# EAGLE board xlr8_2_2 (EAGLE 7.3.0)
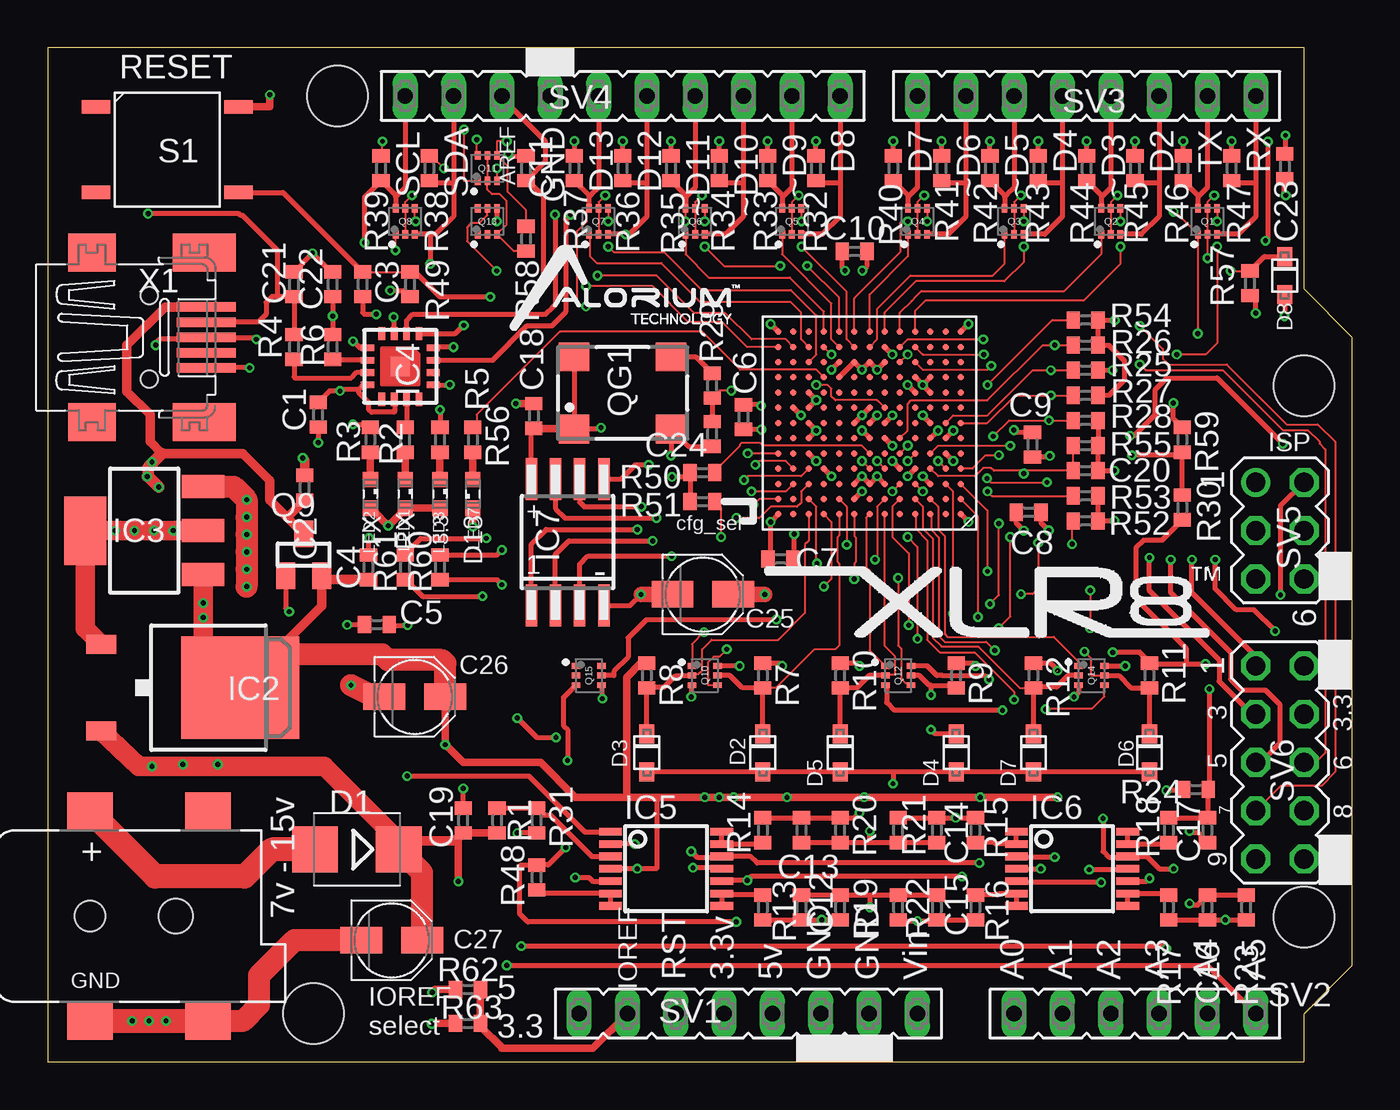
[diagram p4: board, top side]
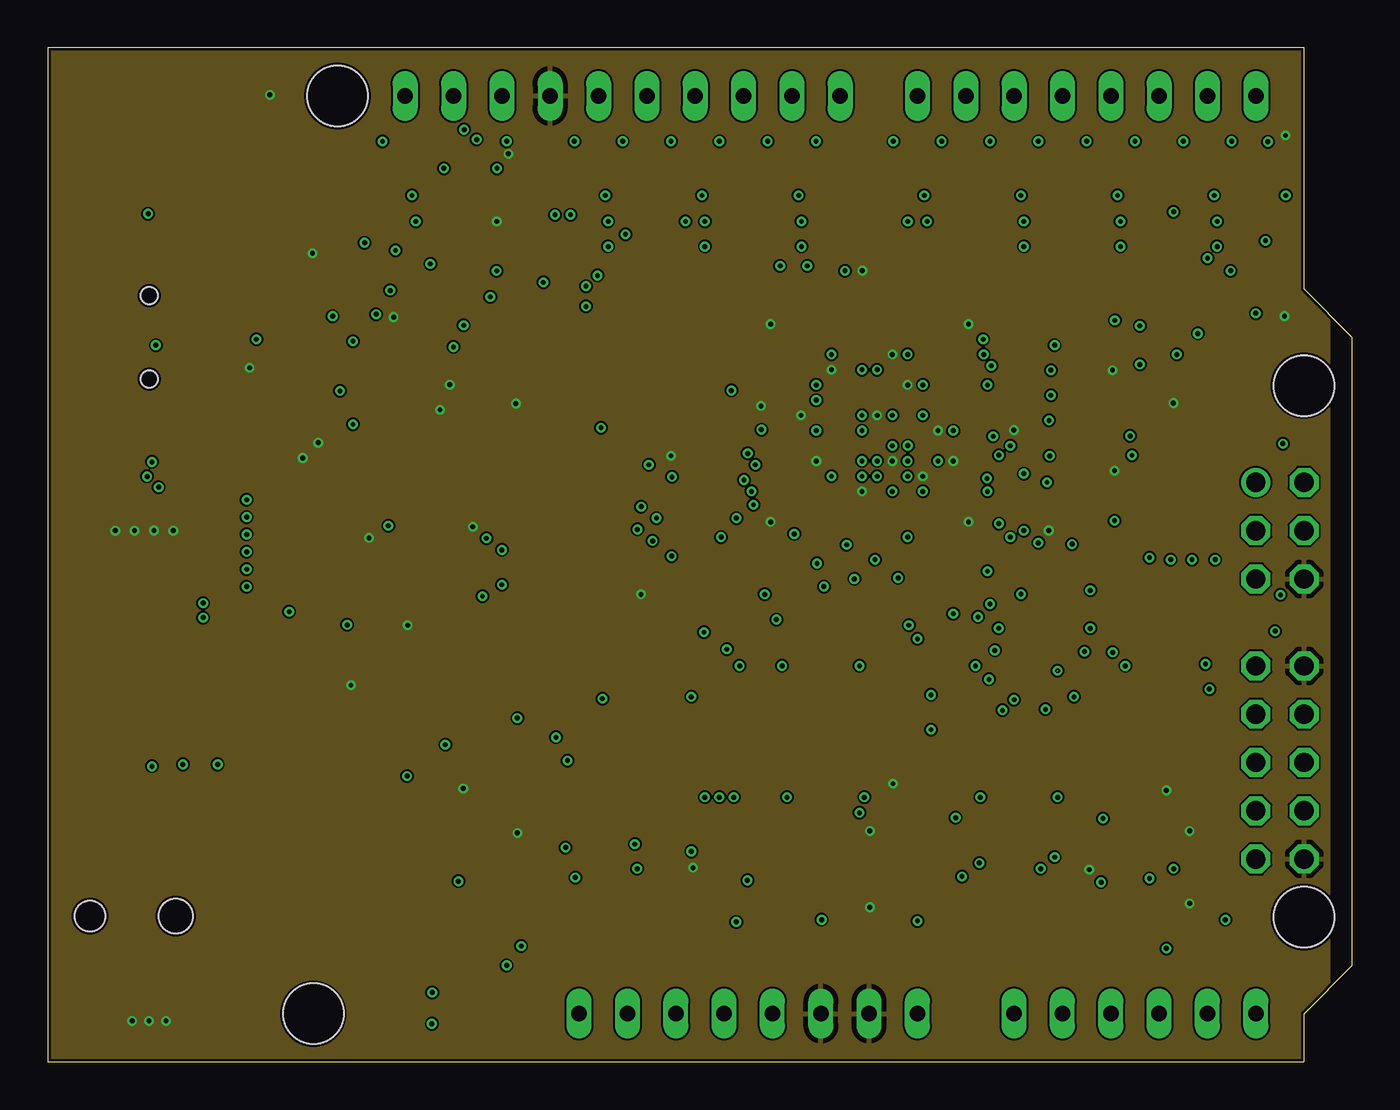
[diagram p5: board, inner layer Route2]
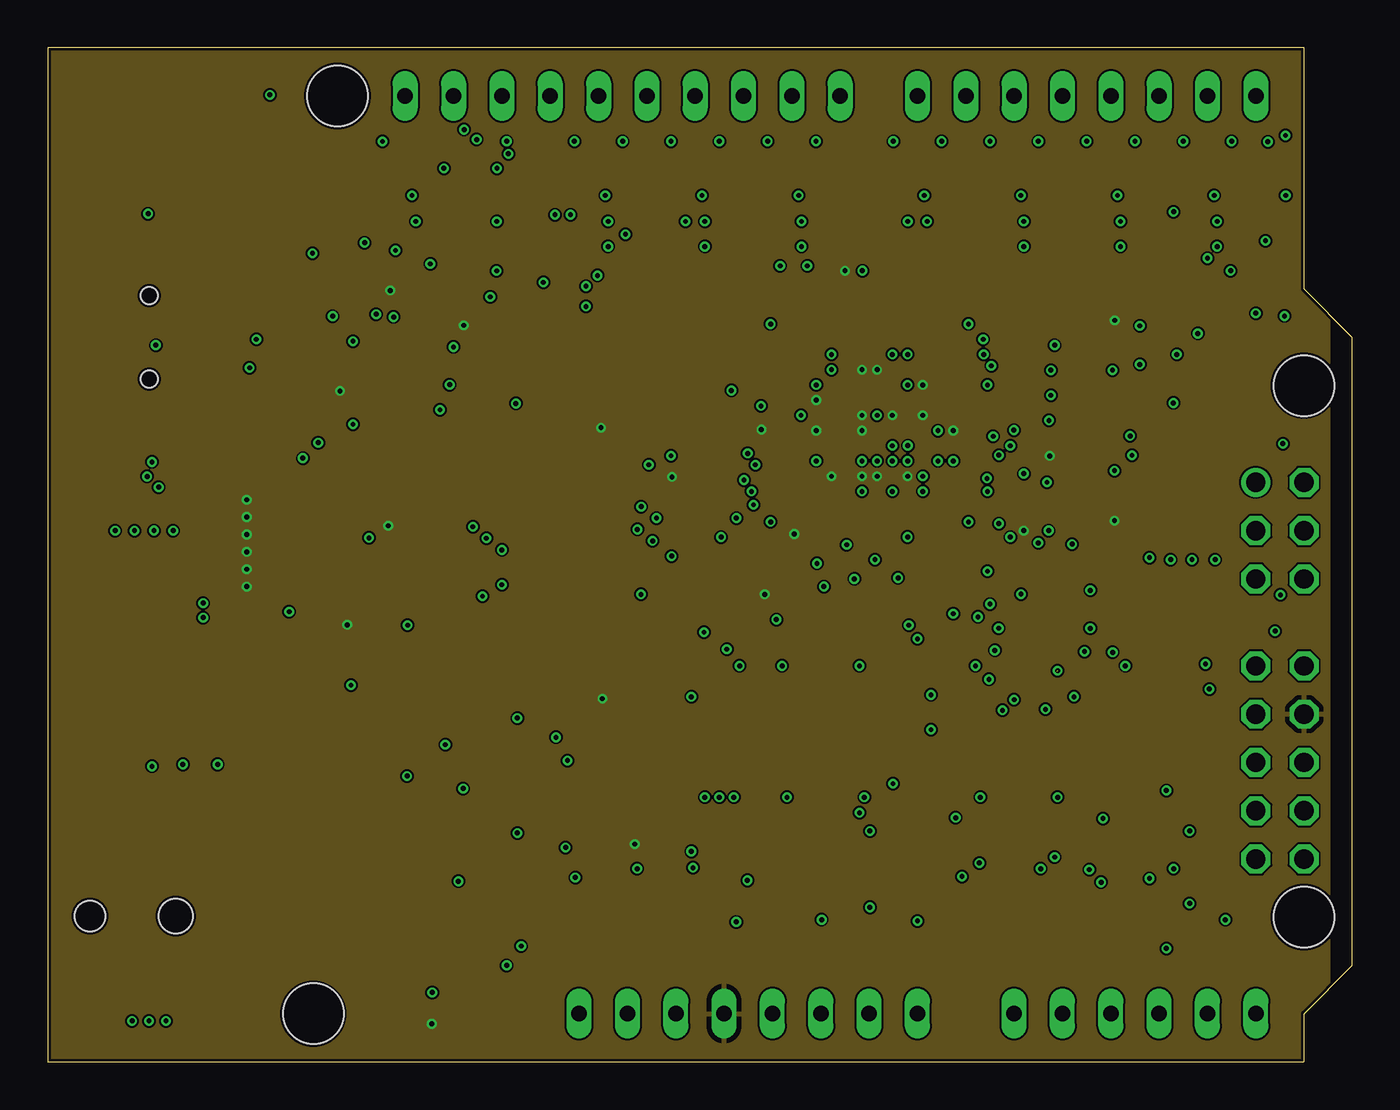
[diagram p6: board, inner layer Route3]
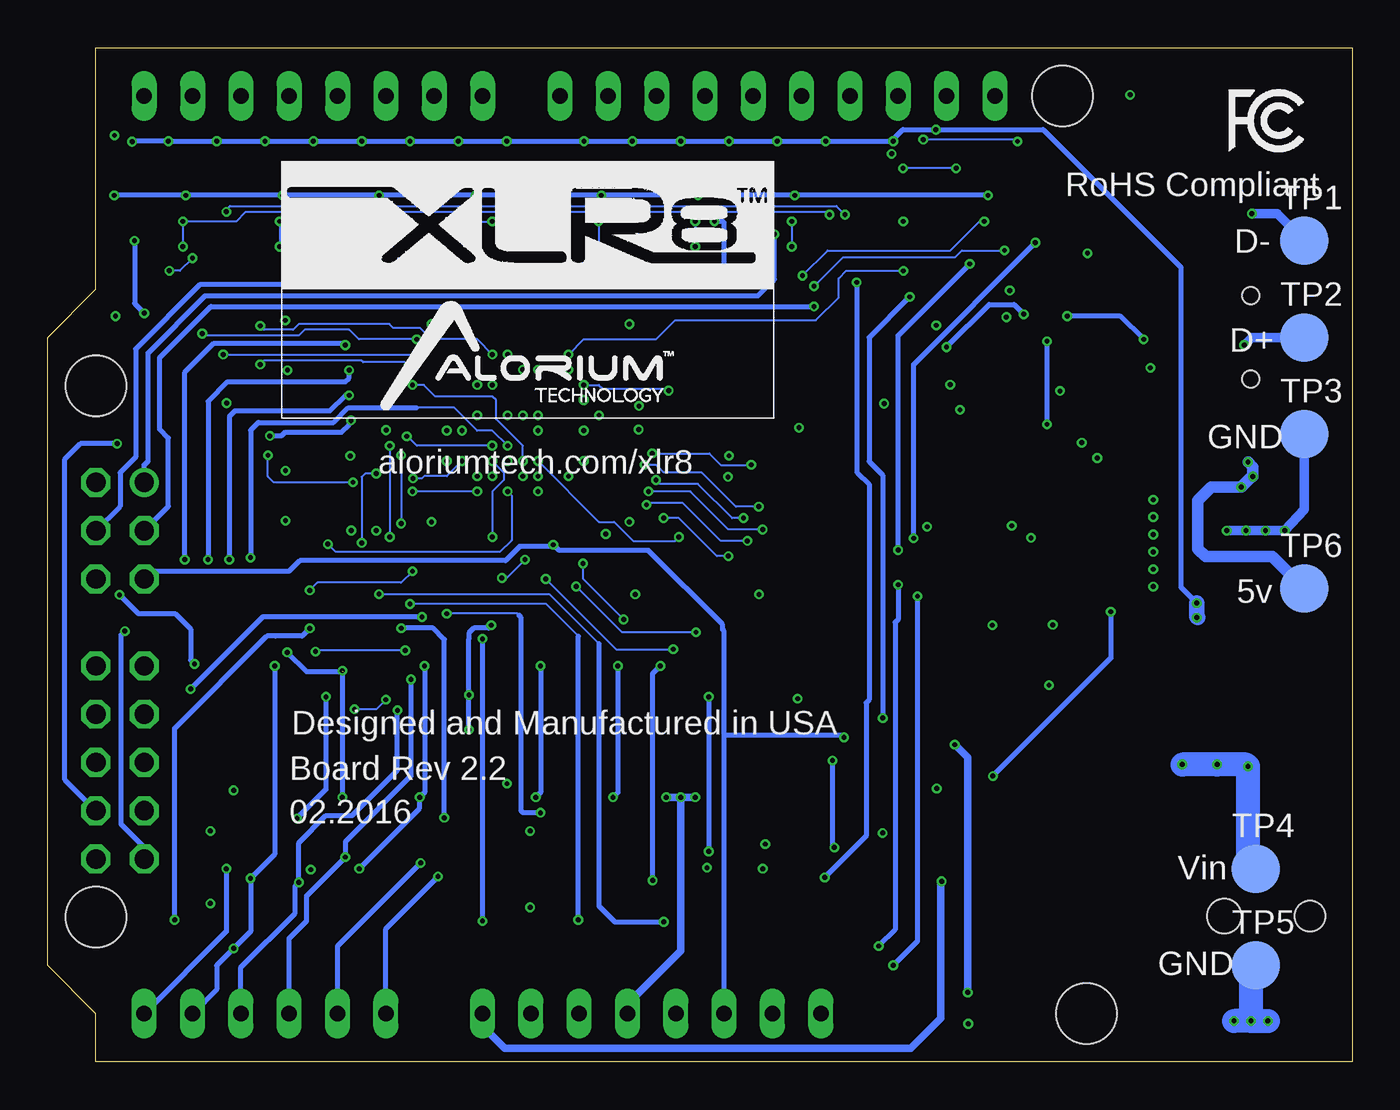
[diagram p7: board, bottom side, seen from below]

Size 68.58 x 53.34 mm. Coordinates in mm from the lower left corner, seen from the top.
Outline: 66.02,0 0,0 0,53.34 66.04,53.34 66.04,40.64 68.58,38.1 68.58,5.08 66.04,2.54 66.04,0
Copper layers (1*2*3*16): Top 0.035mm / dielectric 0.204mm / Route2 0.035mm / dielectric 0.252mm / Route3 0.035mm / dielectric 0.204mm / Bottom 0.035mm
Design rules "default *": minimum track width 4mil, minimum drill 10mil, track to track 4mil, track to pad 5mil, pad to pad 6mil, via to via 6mil, smd to smd 6mil, copper to edge 6mil, drill to drill 6mil, minimum pad ring 10mil, minimum via ring 5mil, stop-mask expansion 0mil, vias tented up to drill 25mil, thermal gap 10mil
Holes 3.17 mm at 15.24,50.8 66.04,7.62 66.04,35.56 13.97,2.54

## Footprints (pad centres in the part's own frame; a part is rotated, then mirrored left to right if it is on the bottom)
C0402 = smd 0.7 x 0.9: 1 -0.65,0; 2 0.65,0
PANASONIC_B = smd 2.2 x 1.4: + 1.6,0; - -1.6,0
DCJACK_2MM_SMT = smd 2.4 x 2: GND 0,-5.5; GNDBREAK 6.2,-5.5; PWR1 0,5.5; PWR2 6.2,5.5 | hole 1.6: 0,0 | hole 1.8: 4.5,0
SMB = smd 2.4 x 2.4: A 2.2,0; C -2.2,0
SOD-323F = smd 1 x 0.8: A -1,0; C 1,0
DPACK = smd 1 x 1.6: 1 -2.28,-4.8; 3 2.28,-4.8 | smd 5.4 x 6.2: 2 0,2.5
SOT223 = smd 1.219 x 2.235: 1 -2.311,-3.099; 2 0,-3.099; 3 2.311,-3.099 | smd 3.6 x 2.2: 4 0,3.099
QFN16 = smd 0.7 x 0.35: 1 -1.725,0.975; 2 -1.725,0.325; 3 -1.725,-0.325; 4 -1.725,-0.975; 9 1.725,-0.975; 10 1.725,-0.325; 11 1.725,0.325; 12 1.725,0.975 | smd 0.35 x 0.7: 5 -0.975,-1.725; 6 -0.325,-1.725; 7 0.325,-1.725; 8 0.975,-1.725; 13 0.975,1.725; 14 0.325,1.725; 15 -0.325,1.725; 16 -0.975,1.725 | smd 1 x 1: TAB 0,0
SSOP14 = smd 0.4 x 1.2: 1 -1.95,-2.925; 2 -1.3,-2.925; 3 -0.65,-2.925; 4 0,-2.925; 5 0.65,-2.925; 6 1.3,-2.925; 7 1.95,-2.925; 8 1.95,2.925; 9 1.3,2.925; 10 0.65,2.925; 11 0,2.925; 12 -0.65,2.925; 13 -1.3,2.925; 14 -1.95,2.925
SO-08M = smd 0.6 x 2.2: 1 -1.905,-3.33; 2 -0.635,-3.33; 3 0.635,-3.33; 4 1.905,-3.33; 5 1.905,3.33; 6 0.635,3.33; 7 -0.635,3.33; 8 -1.905,3.33
LED_SML0603 = smd 0.8 x 0.8: A 0.75,0; C -0.75,0
SOT-563 = smd 0.3 x 0.45: 1 -0.5,-0.674; 2 0,-0.674; 3 0.5,-0.674; 4 0.5,0.674; 5 0,0.674; 6 -0.5,0.674
SUPER-SOT3 = smd 1 x 1.4: 1 -0.95,-1.1; 2 0.95,-1.1; 3 0,1.1
SM77H = smd 1.6 x 1.5: 1 -2.55,-1.9; 2 2.55,-1.9; 3 2.55,1.9; 4 -2.55,1.9
R0402 = smd 0.7 x 0.9: 1 -0.65,0; 2 0.65,0
6MM_SMT = smd 1.5 x 0.7: 1 0,4.5; 2 7.5,4.5; 3 0,0; 4 7.5,0
FE08 = drill 0.813 long: 1 -8.89,0; 2 -6.35,0; 3 -3.81,0; 4 -1.27,0; 5 1.27,0; 6 3.81,0; 7 6.35,0; 8 8.89,0
FE06 = drill 0.813 long: 1 -6.35,0; 2 -3.81,0; 3 -1.27,0; 4 1.27,0; 5 3.81,0; 6 6.35,0
FE10 = drill 0.813 long: 1 -11.43,0; 2 -8.89,0; 3 -6.35,0; 4 -3.81,0; 5 -1.27,0; 6 1.27,0; 7 3.81,0; 8 6.35,0; 9 8.89,0; 10 11.43,0
MA03-2 = drill 1.016: 1 -2.54,-1.27 | drill 1.016 octagon: 2 -2.54,1.27; 3 0,-1.27; 4 0,1.27; 5 2.54,-1.27; 6 2.54,1.27
MA05-2 = drill 1.016 octagon: 1 -5.08,-1.27; 2 -5.08,1.27; 3 -2.54,-1.27; 4 -2.54,1.27; 5 0,-1.27; 6 0,1.27; 7 2.54,-1.27; 8 2.54,1.27; 9 5.08,-1.27; 10 5.08,1.27
B2,54 = smd 2.54 x 2.54: TP 0,0
UBGA_169 = smd 0.34 x 0.34: A1 -9.6,0; A2 -8.8,0; A3 -8,0; A4 -7.2,0; A5 -6.4,0; A6 -5.6,0; A7 -4.8,0; A8 -4,0; A9 -3.2,0; A10 -2.4,0; A11 -1.6,0; A12 -0.8,0; A13 0,0; B1 -9.6,-0.8; B2 -8.8,-0.8; B3 -8,-0.8; B4 -7.2,-0.8; B5 -6.4,-0.8; B6 -5.6,-0.8; B7 -4.8,-0.8; B8 -4,-0.8; B9 -3.2,-0.8; B10 -2.4,-0.8; B11 -1.6,-0.8; B12 -0.8,-0.8; B13 0,-0.8; C1 -9.6,-1.6; C2 -8.8,-1.6; C3 -8,-1.6; C4 -7.2,-1.6; C5 -6.4,-1.6; C6 -5.6,-1.6; C7 -4.8,-1.6; C8 -4,-1.6; C9 -3.2,-1.6; C10 -2.4,-1.6; C11 -1.6,-1.6; C12 -0.8,-1.6; C13 0,-1.6; D1 -9.6,-2.4; D2 -8.8,-2.4; D3 -8,-2.4; D4 -7.2,-2.4; D5 -6.4,-2.4; D6 -5.6,-2.4; D7 -4.8,-2.4; D8 -4,-2.4; D9 -3.2,-2.4; D10 -2.4,-2.4; D11 -1.6,-2.4; D12 -0.8,-2.4; D13 0,-2.4; E1 -9.6,-3.2; E2 -8.8,-3.2; E3 -8,-3.2; E4 -7.2,-3.2; E5 -6.4,-3.2; E6 -5.6,-3.2; E7 -4.8,-3.2; E8 -4,-3.2; E9 -3.2,-3.2; E10 -2.4,-3.2; E11 -1.6,-3.2; E12 -0.8,-3.2; E13 0,-3.2; F1 -9.6,-4; F2 -8.8,-4; F3 -8,-4; F4 -7.2,-4; F5 -6.4,-4; F6 -5.6,-4; F7 -4.8,-4; F8 -4,-4; F9 -3.2,-4; F10 -2.4,-4; F11 -1.6,-4; F12 -0.8,-4; F13 0,-4; G1 -9.6,-4.8; G2 -8.8,-4.8; G3 -8,-4.8; G4 -7.2,-4.8; G5 -6.4,-4.8; G6 -5.6,-4.8; G7 -4.8,-4.8; G8 -4,-4.8; G9 -3.2,-4.8; G10 -2.4,-4.8; G11 -1.6,-4.8; G12 -0.8,-4.8; G13 0,-4.8; H1 -9.6,-5.6; H2 -8.8,-5.6; H3 -8,-5.6; H4 -7.2,-5.6; H5 -6.4,-5.6; H6 -5.6,-5.6; H7 -4.8,-5.6; H8 -4,-5.6; H9 -3.2,-5.6; H10 -2.4,-5.6; H11 -1.6,-5.6; H12 -0.8,-5.6; H13 0,-5.6; J1 -9.6,-6.4; J2 -8.8,-6.4; J3 -8,-6.4; J4 -7.2,-6.4; J5 -6.4,-6.4; J6 -5.6,-6.4; J7 -4.8,-6.4; J8 -4,-6.4; J9 -3.2,-6.4; J10 -2.4,-6.4; J11 -1.6,-6.4; J12 -0.8,-6.4; J13 0,-6.4; K1 -9.6,-7.2; K2 -8.8,-7.2; K3 -8,-7.2; K4 -7.2,-7.2; K5 -6.4,-7.2; K6 -5.6,-7.2; K7 -4.8,-7.2; K8 -4,-7.2; K9 -3.2,-7.2; K10 -2.4,-7.2; K11 -1.6,-7.2; K12 -0.8,-7.2; K13 0,-7.2; L1 -9.6,-8; L2 -8.8,-8; L3 -8,-8; L4 -7.2,-8; L5 -6.4,-8; L6 -5.6,-8; L7 -4.8,-8; L8 -4,-8; L9 -3.2,-8; L10 -2.4,-8; L11 -1.6,-8; L12 -0.8,-8; L13 0,-8; M1 -9.6,-8.8; M2 -8.8,-8.8; M3 -8,-8.8; M4 -7.2,-8.8; M5 -6.4,-8.8; M6 -5.6,-8.8; M7 -4.8,-8.8; M8 -4,-8.8; M9 -3.2,-8.8; M10 -2.4,-8.8; M11 -1.6,-8.8; M12 -0.8,-8.8; M13 0,-8.8; N1 -9.6,-9.6; N2 -8.8,-9.6; N3 -8,-9.6; N4 -7.2,-9.6; N5 -6.4,-9.6; N6 -5.6,-9.6; N7 -4.8,-9.6; N8 -4,-9.6; N9 -3.2,-9.6; N10 -2.4,-9.6; N11 -1.6,-9.6; N12 -0.8,-9.6; N13 0,-9.6
32005-201 = smd 3.1 x 0.5: 1 3,1.6; 2 3,0.8; 3 3,0; 4 3,-0.8; 5 3,-1.6 | smd 2.5 x 2: M1 -3,-4.45; M2 -3,4.45 | smd 3.3 x 2: M3 2.9,4.45; M4 2.9,-4.45 | hole 0.9: 0,2.2; 0,-2.2

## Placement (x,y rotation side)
C1  10uf  [C0402]  14.22,34.04 90 top
C2  10uF  [C0402]  13.52,30.2 90 top
C3  .1uf  [C0402]  16.56,40.89 270 top
C4  10uF  [C0402]  16.87,26.01 90 top
C5  10uF  [C0402]  17.3,23 0 top
C6  .1uF  [C0402]  36.58,33.91 90 top
C7  .1uF  [C0402]  38.52,26.45 180 top
C8  .1uF  [C0402]  51.56,28.91 0 top
C9  .1uF  [C0402]  51.77,32.46 90 top
C10  .1uF  [C0402]  42.42,42.62 0 top
C11  1nf  [C0402]  25.15,46.99 90 top
C12  1nf  [C0402]  39.62,8.13 90 top
C13  1nf  [C0402]  39.62,12.19 270 top
C14  1nf  [C0402]  46.74,12.19 270 top
C15  1nf  [C0402]  46.74,8.13 90 top
C16  1nf  [C0402]  60.96,8.13 90 top
C17  1nf  [C0402]  60.96,12.19 270 top
C18  .1uf  [C0402]  25.56,33.97 90 top
C19  10uF  [C0402]  21.84,12.7 90 top
C20  1nf  [C0402]  54.56,31.09 0 top
C21  47pf  [C0402]  12.95,40.89 90 top
C22  47pf  [C0402]  14.99,40.89 90 top
C23  1nf  [C0402]  65.02,47.09 90 top
C24  47pf  [C0402]  34.92,33.02 270 top
C25  47uf  [PANASONIC_B]  34.44,24.59 0 top
C26  47uf  [PANASONIC_B]  19.3,19.2 0 top
C27  22uf  [PANASONIC_B]  18.08,6.4 0 top
CN2  [DCJACK_2MM_SMT]  2.24,7.67 0 top
D1  [SMB]  16.26,11.18 180 top
D2  [SOD-323F]  37.59,16.26 90 top
D3  [SOD-323F]  31.5,16.26 90 top
D4  [SOD-323F]  47.75,16.26 90 top
D5  [SOD-323F]  41.66,16.26 90 top
D6  [SOD-323F]  57.91,16.26 90 top
D7  [SOD-323F]  51.82,16.26 90 top
D8  [SOD-323F]  65.02,41.35 90 top
IC2  MC33269D-5.0  [DPACK]  7.62,19.68 270 top
IC3  LT1963EST-3.3  [SOT223]  5.08,27.94 90 top
IC4  FT230XQ  [QFN16]  18.54,36.58 270 top
IC5  LM2902PT  [SSOP14]  32.51,10.16 270 top
IC6  LM2902PT  [SSOP14]  53.85,10.16 270 top
IC7  24AA128SM  [SO-08M]  27.33,27.33 0 top
LED1  yellow  [LED_SML0603]  18.8,29.87 270 top
LED2  red  [LED_SML0603]  16.97,29.87 270 top
LED3  green  [LED_SML0603]  20.62,29.87 270 top
LED7  blue  [LED_SML0603]  22.35,29.87 90 top
Q1  EM6K34  [SOT-563]  60.96,44.2 0 top
Q2  EM6K34  [SOT-563]  55.88,44.2 0 top
Q3  EM6K34  [SOT-563]  50.8,44.2 0 top
Q4  EM6K34  [SOT-563]  45.72,44.2 0 top
Q5  EM6K34  [SOT-563]  39.12,44.2 0 top
Q6  EM6K34  [SOT-563]  34.04,44.2 0 top
Q7  EM6K34  [SOT-563]  28.96,44.2 0 top
Q8  EM6K34  [SOT-563]  18.8,44.2 0 top
Q9  FDN360P  [SUPER-SOT3]  13.46,26.67 0 top
Q10  EM6K34  [SOT-563]  34.54,20.32 270 top
Q11  EM6J1T2R  [SOT-563]  23.11,46.99 0 top
Q12  EM6K34  [SOT-563]  44.7,20.32 270 top
Q13  EM6K34  [SOT-563]  23.11,44.2 0 top
Q14  EM6K34  [SOT-563]  54.86,20.32 270 top
Q15  EM6J1T2R  [SOT-563]  28.45,20.32 270 top
QG1  SM77H  [SM77H]  30.23,35.18 0 top
R1  10k  [R0402]  23.62,12.7 270 top
R2  220  [R0402]  18.8,32.72 270 top
R3  220  [R0402]  16.97,32.72 270 top
R4  22  [R0402]  12.95,37.59 90 top
R5  220  [R0402]  20.62,32.72 270 top
R6  22  [R0402]  14.99,37.59 90 top
R7  280  [R0402]  37.59,20.32 270 top
R8  280  [R0402]  31.5,20.32 270 top
R9  280  [R0402]  47.75,20.32 270 top
R10  280  [R0402]  41.66,20.32 270 top
R11  280  [R0402]  57.91,20.32 270 top
R12  280  [R0402]  51.82,20.32 270 top
R13  1.7k  [R0402]  37.59,8.13 270 top
R14  1.7k  [R0402]  37.59,12.19 90 top
R15  1.7k  [R0402]  48.77,12.19 90 top
R16  1.7k  [R0402]  48.77,8.13 270 top
R17  1.7k  [R0402]  58.93,8.13 270 top
R18  1.7k  [R0402]  58.93,12.19 90 top
R19  3.3k  [R0402]  41.66,8.13 270 top
R20  3.3k  [R0402]  41.66,12.19 90 top
R21  3.3k  [R0402]  44.7,12.19 90 top
R22  3.3k  [R0402]  44.7,8.13 270 top
R23  3.3k  [R0402]  62.99,8.13 270 top
R24  3.3k  [R0402]  60.35,14.33 0 top
R25  1k  [R0402]  54.56,36.37 180 top
R26  10k  [R0402]  54.56,37.69 0 top
R27  10k  [R0402]  54.56,35.05 0 top
R28  1k  [R0402]  54.56,33.73 0 top
R29  22  [R0402]  34.92,35.56 90 top
R30  1.7k  [R0402]  59.64,29.16 90 top
R31  10k  [R0402]  25.7,12.7 90 top
R32  1k  [R0402]  40.39,46.99 270 top
R33  1k  [R0402]  37.85,46.99 270 top
R34  1k  [R0402]  35.31,46.99 270 top
R35  1k  [R0402]  32.77,46.99 270 top
R36  1k  [R0402]  30.23,46.99 270 top
R37  1k  [R0402]  27.69,46.99 270 top
R38  1k  [R0402]  20.07,46.99 270 top
R39  1k  [R0402]  17.53,46.99 270 top
R40  1k  [R0402]  44.45,46.99 90 top
R41  1k  [R0402]  46.99,46.99 90 top
R42  1k  [R0402]  49.53,46.99 90 top
R43  1k  [R0402]  52.07,46.99 90 top
R44  1k  [R0402]  54.61,46.99 90 top
R45  1k  [R0402]  57.15,46.99 90 top
R46  1k  [R0402]  59.69,46.99 90 top
R47  1k  [R0402]  62.23,46.99 90 top
R48  1.7k  [R0402]  25.7,9.7 90 top
R49  5k  [R0402]  19.05,40.89 270 top
R50  5k  [R0402]  34.42,30.99 180 top
R51  5k  [R0402]  34.42,29.46 180 top
R52  1k  [R0402]  54.56,28.45 0 top
R53  1k  [R0402]  54.56,29.77 0 top
R54  220  [R0402]  54.56,39.01 0 top
R55  3.3k  [R0402]  54.56,32.41 180 top
R56  220  [R0402]  22.35,32.72 90 top
R57  280  [R0402]  63.2,40.94 90 top
R58  5k  [R0402]  25.15,43.28 270 top
R59  3.3k  [R0402]  59.64,32.72 270 top
R60  0 ohm  [R0402]  20.62,26.01 90 top
R61  0 ohm  [R0402]  18.8,26.01 90 top
R62  0  [R0402]  22.1,3.81 180 top
R63  0  [R0402]  22.1,2.03 0 top
S1  RDT1034SMT  [6MM_SMT]  2.54,45.72 0 top
SV1  [FE08]  36.83,2.54 0 top
SV2  [FE06]  57.15,2.54 0 top
SV3  [FE08]  54.61,50.8 180 top
SV4  [FE10]  30.23,50.8 180 top
SV5  [MA03-2]  64.77,27.94 270 top
SV6  [MA05-2]  64.77,15.75 270 top
TP1  TPB2,54  [B2,54]  2.54,43.18 0 bottom
TP2  TPB2,54  [B2,54]  2.54,38.1 0 bottom
TP3  TPB2,54  [B2,54]  2.54,33.02 0 bottom
TP4  TPB2,54  [B2,54]  5.08,10.16 0 bottom
TP5  TPB2,54  [B2,54]  5.08,5.08 0 bottom
TP6  TPB2,54  [B2,54]  2.54,24.89 0 bottom
U1  [UBGA_169]  38.4,28.8 180 top
X1  MINI-USB-32005-201  [32005-201]  5.33,38.1 0 top

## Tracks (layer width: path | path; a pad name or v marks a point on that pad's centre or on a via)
3.3V  (via drill 0.25, 0.25 pad 0.51)
  Top 0.102: R27.2 55.21,35.11
  Top 0.254: U1.J11 v40.4,34.8 U1.H11 | U1.G11 v40.4,33.2 U1.F11 | U1.L6 v43.6,36.4 U1.L7 v42.8,36.4 U1.L8 U1.K9 | U1.C8 v42.8,30.8 U1.C7 v43.6,30.8 U1.C6 | U1.K3 v46,35.6 | U1.J3 v46,35.6 | U1.K4 v46,35.6 | U1.H7 v42.8,34 U1.G8 | U1.D4 v45.2,30.8 | U1.F2 v47.6,33.2 | U1.G6 v44.4,34 | U1.F7 v42.8,33.2 | U1.D10 v41.2,30.8 | QG1.4 QG1.1 29.01,33.28 v29.08,33.35 | U1.G3 v46,34 | R53.2 R52.2 55.22,28.46 v56.07,28.46 | IC4.1 21.43,38.3 v21.87,38.74 | v18.01,40.57 18.73,40.57 R49.2 | IC4.8 16.6,35.6 16.36,35.36 | 16.36,35.36 15.44,35.36 v15.37,35.28 14.82,35.28 C1.2 | v30.86,11.46 IC5.2 | R50.2 33.74,30.96 | 33.74,30.96 33.77,30.94 R51.2 | 17.13,28.97 LED2.A | 18.68,28.97 LED1.A | v41.91,41.6 41.77,41.75 C10.1 | v52.67,31.87 52.61,31.81 C9.1 | C7.1 39.24,26.53 v39.24,27.76 | C5.1 16.64,22.99 v15.75,22.99 | v37.52,33.25 37.51,33.26 C6.1 | IC4.10 18.24,34.83 18.24,34.19 18.21,34.16 17.02,34.16 16.89,34.29 16.89,34.67 16.36,35.2 16.36,35.36 | IC3.3 8.21,30.28 | v56.09,38.99 56.07,39.01 R54.2 R26.2 55.78,37.69 56.59,36.88 56.59,35.87 55.78,35.05 R27.2 | v51.31,27.94 50.91,28.34 C8.1 | IC7.8 25.43,33.18 C18.1 | 33.74,30.96 33.54,30.76 v32.82,30.76 | Q15.4 29.12,19.14 v29.16,19.1
  Top 0.406: C18.1 27.64,33.32 QG1.1 | 17.13,28.97 v17.91,28.19 18.68,28.97 | LED3.A LED1.A | R63.1 20.22,2.03 v20.19,2.01
  Top 0.813: C25.+ v37.69,24.59
  Top 1.168: IC3.3 9.78,30.25 v10.46,29.57 v10.46,28.65 v10.46,27.74 v10.46,26.82 v10.46,25.91 v10.46,24.99
  pour Route3: 0,53.2 0,0 67.4,0 67.4,53.2
5V  (via drill 0.25)  (1 unrouted)
  Top 0.102: R58.1 25.15,44.78 24.18,45.75 24.18,47.09 Q11.4 23.61,48.41 v24.13,48.41 | Q11.1 21.89,46.32 v21.89,49.02
  Top 0.254: R47.2 v62.23,48.41 | v27.69,48.41 R37.1 | R46.2 v59.69,48.41 | R45.2 v57.15,48.41 | R44.2 v54.61,48.41 | R43.2 v52.07,48.41 | R42.2 v49.53,48.41 | R41.2 v46.99,48.41 | R40.2 v44.45,48.41 | R32.1 v40.39,48.41 | R33.1 v37.85,48.41 | R34.1 v35.31,48.41 | R35.1 v32.77,48.41 | R36.1 v30.23,48.41 | IC5.4 v30.99,10.16 32,10.16 32,13.89 32.03,13.92 | R7.1 38.47,20.97 v38.61,20.83 | R10.1 42.53,20.97 v42.67,20.83 | R9.1 48.63,20.97 v48.77,20.83 | R12.1 52.69,20.97 v53.09,20.57 | R11.1 57.93,20.95 | v64.14,48.39 64.14,43.31 v64.01,43.18 | v63.5,39.37 63.5,39.99 R57.1 | IC6.4 v52.2,10.16 | 58.05,20.83 R11.1 | 58.01,20.93 57.95,20.93 R11.1 | 58.01,20.93 57.4,21.54 v55.98,21.54 | 58.01,20.93 59.84,20.93 | 59.84,20.93 v60.86,20.93 | R30.1 58.56,27.43 57.61,27.43 57.2,27.03 57.2,24.38 59.84,21.74 59.84,20.93 | SV5.2 64.8,29.23 v64.8,24.56
  Top 0.406: R8.1 31.18,20.97 30.43,20.22 30.43,13.97 30.48,13.92 | v53.09,13.92 v49.02,13.92 v42.93,13.92 v38.86,13.92 v36.07,13.92 v35.31,13.92 v34.54,13.92 32.03,13.92 30.48,13.92 | C26.+ v20.9,16.69 21.84,15.75 25.91,15.75 27.74,13.92 30.48,13.92 | R62.2 20.37,3.81 v20.22,3.66
  Top 0.508: C4.1 14.62,25.36 Q9.2 14.41,23.98 IC2.2 8.18,21.63
  Top 1.016: IC3.1 v8.18,24.13 v8.18,23.37 8.18,21.63
  Top 1.168: C26.+ 20.9,20.95 20.73,21.13 17.88,21.13 17.58,21.44 11.87,21.44 IC2.2
  Bottom 0.254: v38.61,20.83 38.61,14.17 v38.86,13.92 | v42.67,20.83 42.67,14.17 v42.93,13.92 | v48.77,20.83 48.77,14.17 v49.02,13.92 49.02,13.34 v52.2,10.16 | v53.09,20.57 v53.09,13.92 | v64.14,48.39 64.11,48.41 v62.23,48.41 v59.69,48.41 v57.15,48.41 v54.61,48.41 v52.07,48.41 v49.53,48.41 v46.99,48.41 v44.45,48.41 v40.39,48.41 v37.85,48.41 v35.31,48.41 v32.77,48.41 v30.23,48.41 v27.69,48.41 v24.13,48.41 24.13,48.51 23.62,49.02 v21.89,49.02 16.26,49.02 9.02,41.78 9.02,24.97 v8.18,24.13 v8.18,23.37 | v64.01,43.18 64.01,39.88 v63.5,39.37 | v55.98,21.54 54.97,20.52 53.03,20.52 | v60.86,20.93 61.06,21.13 61.06,22.76 61.87,23.57 63.8,23.57 v64.8,24.56
  Bottom 0.406: SV1.5 38.1,3.05 35.31,5.84 v35.31,13.92 | v20.22,3.66 20.22,16 v20.9,16.69 | v35.31,13.92 v36.07,13.92 | v35.31,13.92 v34.54,13.92
  Bottom 0.813: v8.18,24.13 8.18,23.42 8.13,23.37
ANA_CMP_REF
  Top 0.254: SV3.7 48.26,46.23 | 48.26,46.23 48.26,44.45 47.33,43.52 Q4.3 | R41.1 47.1,46.23 48.26,46.23
ANA_UP  (via drill 0.25)
  Top 0.102: v40.44,26.21 40.4,26.25 40.4,29.2 U1.B11
  Top 0.254: 31.48,23.27 31.48,23.26 | 31.48,23.26 v38.3,23.27 | 31.48,23.26 30.52,22.3 30.52,21.27 29.77,20.52 29.77,20.32 Q15.5
  Bottom 0.102: v38.3,23.27 40.44,25.4 v40.44,26.21
AREF  (via drill 0.25)
  Top 0.102: C11.1 25.24,46.34 | 29.58,9.5 IC5.5
  Top 0.254: SV4.8 23.88,50.7 26.16,48.41 26.16,47.36 C11.1 | 25.24,46.34 26.06,45.52 v26.06,41 | v27.74,9.7 28.45,9.7 28.65,9.5 29.58,9.5
  Bottom 0.254: v27.74,9.7 25.55,11.89 25.55,18.89 25.4,19.04 25.4,30.38 26.03,31 26.03,40.96 v26.06,41
AREF_SCALED  (via drill 0.25)
  Top 0.102: R55.2 C20.1 51.31,31.09 | v52.07,27.3 52.07,24.9 51.77,24.6 v51.16,24.6 | 25.69,10.36 R48.2 | U1.D3 46.8,30.8 48.75,30.8 | 48.77,30.79 48.75,30.8 | 51.31,31.09 49.73,31.09 49.58,31.24 49.17,31.24 48.75,30.82 48.75,30.8 | 51.31,31.09 v51.31,30.94
  Top 0.254: 25.69,10.36 24.89,10.36 24.81,10.28 24.81,7.8 25.24,7.37 v36.2,7.37 | v27.33,15.85 27.33,17.48 27.13,17.68 27.13,19.17 Q15.3 | v27.23,11.28 26.3,10.35 R48.2
  Bottom 0.102: v52.07,27.3 52.07,30.76 51.89,30.94 v51.31,30.94 | v51.16,24.6 42.2,24.6 39.6,22
  Bottom 0.254: 39.6,22 39.6,8.2 38.77,7.37 v36.2,7.37 | v27.33,15.85 27.33,11.38 v27.23,11.28
DIG_IO_0  (via drill 0.25)
  Top 0.102: v34.5,22.6 33.87,21.97 Q10.1 | U1.A10 41.2,28.4 41.2,25.4 v40.8,25
  Bottom 0.102: v40.8,25 38.4,22.6 v34.5,22.6
DIG_IO_0_OE
  Top 0.102: 31.66,19.87 31.82,19.71 | Q10.2 33.95,20.4 34.2,20.4 34.4,20.6 34.4,21.7 34.9,22.2 38.4,22.2 39.8,23.6 39.8,27.2 40,27.4 U1.A11
  Top 0.254: D3.C R8.2 31.66,19.87 | 31.82,19.71 32.41,19.71 33.02,20.32 Q10.2
DIG_IO_1  (via drill 0.25)
  Top 0.102: U1.A8 42.4,27.65 42.47,27.58 42.47,26.28 42.4,26.21 v42.4,25.4 | v35.7,21.7 35.3,21.3 35,21.3 34.7,21 34.7,19.8 34.72,19.82 Q10.4
  Bottom 0.102: v42.4,25.4 38.7,21.7 v35.7,21.7
DIG_IO_1_OE
  Top 0.102: U1.A9 41.6,27.68 | R7.2 38.27,19.67 40.3,21.7 41.4,21.7 41.6,21.9 41.6,26.21 41.5,26.3 41.5,27.58 41.6,27.68 | 41.6,27.68
  Top 0.254: D2.C R7.2 36.52,19.67 35.87,20.32 Q10.5
DIG_IO_2
  Top 0.102: Q12.1 43.2,21.65 43.2,25.84 43.03,26.01 43.03,28.63 U1.A7
DIG_IO_2_OE
  Top 0.102: Q12.2 44.08,20.37 44.5,20.37 44.55,20.42 44.55,21.34 44,21.89 U1.A6
  Top 0.254: D5.C R10.2 42.53,19.67 43.18,20.32 Q12.2
DIG_IO_3  (via drill 0.25)
  Top 0.102: U1.B6 43.6,29.2 43.6,26.53 v43.48,26.42 | Q12.4 45.28,19.91 45.11,19.91 44.86,20.17 44.86,21.74 44.7,21.89 v44.7,25.45
  Bottom 0.102: v44.7,25.45 44.45,25.45 v43.48,26.42
DIG_IO_3_OE  (via drill 0.25)
  Top 0.102: 46.33,19.81 46.43,19.81 | 47.61,19.81 R9.2 | U1.B5 44.4,29.2 44.4,27.6 45.26,26.74 v45.26,22.96
  Top 0.254: 47.61,19.81 46.43,19.81 v46.43,19.3 | D4.C 46.65,17.26 v46.43,17.48 | 46.33,19.81 45.82,20.32 Q12.5
  Bottom 0.254: v46.43,17.48 v46.43,19.3 46.43,22.25 46.43,22.55 46.18,22.81 45.41,22.81 v45.26,22.96
DIG_IO_4
  Top 0.102: U1.B3 46.8,29.2 46.8,28 47.14,27.66 47.14,22.5 47.3,22.35 52.88,22.35 54.19,21.05 Q14.1
DIG_IO_4_OE
  Top 0.102: 51.86,19.71 R12.2 51.09,19.67 48.92,21.84 46.99,21.84 46.53,22.3 46.53,27.52 46,28.05 46,29.2 U1.B4
  Top 0.254: Q14.2 53.65,20.32 53.03,19.71 51.86,19.71 | R12.2 D7.C
DIG_IO_5  (via drill 0.25)
  Top 0.102: U1.A4 45.62,28.78 45.62,28.04 46.23,27.43 46.23,22.2 46.89,21.54 48.72,21.54 50.8,19.46 v50.8,19.05 | 55.54,19.52 Q14.4 55.54,19.22 54.91,18.59 52.5,18.59 v52.45,18.54
  Bottom 0.102: v50.8,19.05 51.31,18.54 v52.45,18.54
DIG_IO_5_OE  (via drill 0.25)
  Top 0.102: U1.A3 46.43,28.77 46.43,27.99 46.84,27.58 46.84,22.4 47.14,22.1 49.33,22.1 v49.78,21.64 | Q14.5 54.86,20.32 54.86,21.21 v54.5,21.58
  Top 0.254: Q14.5 56.29,20.32 56.94,19.67 R11.2 D6.C
  Bottom 0.102: v49.78,21.64 54.43,21.64 v54.5,21.58
GND  (via drill 0.25, 0.25 pad 0.51)
  Top 0.254: U1.N13 v38,38.8 | U1.L9 v41.2,36.4 | U1.M6 v44.4,37.2 | U1.A13 v38,28.4 38,26.59 C7.2 | U1.A1 v48.4,28.4 | U1.J4 v45.2,35.6 | U1.F3 v46.8,33.2 | U1.G7 v43.6,34 | U1.E2 v47.6,31.6 | U1.E11 v40.4,31.6 | U1.H12 v39.6,34 | U1.B8 v42.8,30 | U1.D5 v44.4,31.6 | U1.C3 v46,30.8 | U1.N1 v48.4,38.8 | v56.07,31.09 C20.2 R55.1 R28.2 | R25.1 v55.97,36.38 | D8.A 65.01,40.34 v65.01,39.22 | C23.2 65.06,47.78 v65.06,48.72 | C12.2 R19.1 43.23,8.78 | C15.2 R22.1 43.23,8.78 | C14.2 R21.1 43.21,11.54 | C13.2 R20.1 43.21,11.54 | R23.1 C16.2 60.96,8.76 60.45,8.26 60.1,8.26 v60.02,8.33 | D6.A D7.A D4.A 44.44,15.26 | 44.44,15.26 D5.A D2.A D3.A | IC5.11 35.38,10.21 v33.92,10.21 | IC6.11 56.73,10.11 v54.75,10.11 | 43.21,11.54 43.22,11.55 v43.22,12.14 | 43.23,8.78 43.22,8.77 v43.22,8.13 | 44.44,15.26 v44.44,14.63 | Q13.4 v23.61,44.2 | 25.13,47.65 C11.2 24.33,47.64 v24.22,47.76 | IC4.3 18.22,39.14 v18.19,39.17 | IC4.13 v21.12,35.6 v21.13,35.61 | C1.1 v14.22,32.57 v14.23,32.57 | C19.2 v21.84,14.38 v21.85,14.38 | R31.1 v24.7,12.05 v24.69,12.04 | CN2.GNDBREAK 7.12,2.17 7.11,2.16 v6.22,2.16 | C24.2 33.69,32.37 QG1.2 32.77,33.27 v32.77,31.88 | v16.89,27.56 16.87,27.53 C4.2 | v60.02,12.14 60.1,12.06 60.45,12.06 60.96,11.56 C17.2 | C21.2 12.95,41.56 v13.92,42.52 14.9,41.54 C22.2 | v10.62,36.5 X1.5 | v42.83,41.61 43.07,41.85 C10.2 | v50.79,33.23 50.9,33.11 C9.2 | C5.2 17.99,22.96 v18.93,22.96 | v37.49,34.5 37.43,34.56 C6.2 | IC3.2 | v20.63,34.29 R5.1 | R24.1 59.65,14.28 v58.8,14.28 | v52.62,27.94 52.21,28.35 C8.2 | R59.1 59.17,33.84 v59.17,34.65 | IC7.4 30.6,24 v31.19,24.59
  Top 0.406: S1.2 11.69,50.22 v11.69,50.85 | v24.61,34.62 C18.2 | LED7.C v22.35,28.14
  Top 0.508: C2.2 13.52,31.65 v13.41,31.75
  Top 0.813: C25.- v31.19,24.59
  Top 1.016: IC2.1 1.98,22.8 IC3.4 v3.56,27.94 6.5,27.94 | IC3.2 v6.6,27.94
  Top 1.168: C26.- 17.17,19.2 v15.95,19.81 | C27.- 12.97,6.4 11.12,4.56 11.12,3 10.3,2.17 CN2.GNDBREAK
  Top 1.27: CN2.GND CN2.GNDBREAK
  Bottom 0.508: TP3.TP 2.54,29.06 v3.56,27.94 v5.59,27.94 | v5.59,27.94 v6.6,27.94
  Bottom 1.27: TP5.TP 5.33,4.72 v5.33,2.16 | v5.33,2.16 v6.22,2.16 | v5.33,2.16 v4.45,2.16
  other vias: 4.57,27.94
  pour Route2: 0,53.2 0,-0.2 67.4,-0.2 67.4,53.2 0.2,53.2
I2C_ENABLE  (via drill 0.25)
  Top 0.102: U1.M10 v41.2,37.2 | Q13.5 23.11,44.51 22.69,44.09 22.25,44.09 22.05,43.89 22.05,43.15 v23.6,41.6
  Bottom 0.102: v41.2,37.2 40.4,38 36.6,38 35.6,39 28.2,39 27,40.2 27,41.2 26.6,41.6 v23.6,41.6
JT6  (via drill 0.25)
  Top 0.102: U1.L4 46,36.4 49.4,36.4 v49.6,36.6 | v57.4,36.68 57.71,36.37 61.77,36.37 64.92,33.22 66.24,33.22 66.85,32.61 66.85,32.51 67.16,32.21 67.16,16.26 66.65,15.75 SV6.6
  Bottom 0.102: v49.6,36.6 49.8,36.8 52,36.8 52.08,36.88 57.2,36.88 v57.4,36.68
JT7  (via drill 0.25)
  Top 0.102: U1.L5 v45.2,37.2 | v57.4,38.71 58.62,37.49 58.62,36.98 58.93,36.68 61.98,36.68 65.13,33.53 66.75,33.53 67.67,32.61 67.67,15.24 66.95,14.53 64.82,14.53 SV6.7
  Bottom 0.102: v45.2,37.2 46,38 48.4,38 49,38.6 50.4,38.6 50.61,38.81 55.37,38.81 55.68,38.51 57.2,38.51 v57.4,38.71
N$1  (via drill 0.25)
  Top 0.102: U1.E5 v45.21,32.41 | v49.7,32.9 50.53,33.73 v52.63,33.73 R28.1
  Top 0.254: v56.9,32.92 57.1,32.92 58.22,34.04 58.22,35.36 58.83,35.97 61.47,35.97 v64.92,32.51
  Bottom 0.102: v45.21,32.41 49.17,32.41 49.66,32.9 v49.7,32.9
  Bottom 0.254: v52.63,33.73 52.73,33.53 53.14,33.12 56.08,33.12 56.29,32.92 v56.9,32.92 | SV6.8 67.67,14.83 67.67,31.7 66.85,32.51 v64.92,32.51
N$2  (via drill 0.25)
  Top 0.102: U1.G1 49.4,33.6 50.85,35.05 v52.73,35.05 R27.1
  Top 0.254: v59.03,26.42 59.03,24.69 62.18,21.54 62.18,20.12 62.74,19.56 64.01,19.56 64.77,18.8 64.77,16.76 63.75,15.75 SV6.5
  Bottom 0.254: v52.73,35.05 52.93,35.05 53.75,34.24 58.73,34.24 59.03,33.93 v59.03,26.42
N$3  (via drill 0.25)
  Top 0.102: U1.G2 47.6,34 49.4,34 51.77,36.37 v52.73,36.37 R25.2
  Top 0.254: v60.15,26.42 60.15,24.69 63.5,21.34 SV6.1
  Bottom 0.254: v52.73,36.37 52.73,35.97 52.93,35.76 59.13,35.76 60.15,34.75 v60.15,26.42
N$4  (via drill 0.25)
  Top 0.102: U1.F5 45.2,33.2 45.2,34.6 45.4,34.8 49.4,34.8 52.29,37.69 v52.93,37.69 R26.1
  Top 0.254: v64.52,22.66 63.4,23.77 62.48,23.77 61.37,24.89 v61.37,26.42
  Bottom 0.254: v61.37,26.42 61.37,36.27 59.84,37.8 53.03,37.8 v52.93,37.69 | SV6.9 63.5,11.28 64.72,12.5 64.72,22.45 v64.52,22.66
N$5  (via drill 0.25)
  Top 0.254: U1.F6 v44.4,32.4 | v57.91,26.52 57.91,24.79 61.57,21.13 61.57,20.02 63.3,18.29 SV6.3
  Bottom 0.102: v44.4,32.4 45.2,33.2 46,33.2 47.2,34.4 49.2,34.4
  Bottom 0.254: 49.2,34.4 52.77,34.4 53.54,33.63 57.51,33.63 57.91,33.22 v57.91,26.52
N$6  (via drill 0.25)
  Top 0.254: R4.2 C21.1 12.09,40.24 | 12.09,40.24 11.8,40.24 11.48,39.93 11.48,39.32 11.07,38.91 8.35,38.91 X1.2 | 12.09,40.24 12.09,42.67 10.26,44.5 10.16,44.5 10.06,44.6 v5.28,44.6
  Bottom 0.254: 2.44,42.67 TP1.TP
  Bottom 0.508: TP1.TP 3.96,44.6 v5.28,44.6
N$7  (via drill 0.25)
  Top 0.254: C22.1 v14.99,39.22 R6.2 | v10.97,38 10.87,38.1 X1.3 8.23,38 5.89,38 5.69,37.8 v5.69,37.69
  Bottom 0.254: v10.97,38 12.19,39.22 v14.99,39.22
  Bottom 0.508: v5.69,37.69 5.28,38.1 TP2.TP
N$8
  Top 0.102: 35.52,8.78 IC5.9
  Top 0.254: R13.1 35.52,8.78 | IC5.9 IC5.8
N$9
  Top 0.102: 37.51,11.46 R14.1
  Top 0.254: 37.51,11.46 IC5.13 IC5.14
N$10
  Top 0.102: 50.92,11.54 50.86,11.48
  Top 0.254: IC6.2 50.92,11.54 IC6.1 | 50.86,11.48 49.78,11.48 49.72,11.54 R15.1
N$11
  Top 0.102: IC6.6 50.92,8.88 50.88,8.84
  Top 0.254: IC6.6 IC6.7 | 50.88,8.84 49.99,8.84 49.93,8.78 R16.1
N$12
  Top 0.102: 58.93,8.86 R17.1
  Top 0.254: 58.93,8.86 IC6.9 IC6.8
N$13
  Top 0.102: 58.93,11.46 R18.1
  Top 0.254: 58.93,11.46 IC6.13 IC6.14
N$14  (via drill 0.25)
  Top 0.102: v49.53,24.08 50,24.55 v50,28.31 | U1.D1 48.6,31.2 49.31,31.91 v50,31.91
  Top 0.254: R13.2 C12.1 v40.69,7.48 R19.2
  Bottom 0.102: v50,31.91 v50,28.31 | 40.69,22.4 42.37,24.08 v49.53,24.08
  Bottom 0.254: v40.69,7.48 40.69,22.4
N$15  (via drill 0.25)
  Top 0.102: U1.C2 47.6,30 47.6,23.67 v47.6,23.57
  Top 0.254: R14.2 C13.1 R20.2 42.41,12.84 v42.67,13.11
  Bottom 0.102: 43.81,23.5 43.89,23.57 v47.6,23.57
  Bottom 0.254: v42.67,13.11 43.59,13.11 43.69,13.21 43.69,23.37 43.81,23.5
N$16
  Top 0.406: R2.2 LED1.C
N$17  (via drill 0.25)
  Top 0.102: U1.E3 46.8,32.4 v50.6,32.4 | v49.99,22.81 50.6,23.42 v50.6,27.6
  Top 0.254: R21.2 C14.1 v47.73,12.84 R15.2
  Bottom 0.102: v50.6,32.4 v50.6,27.6
  Bottom 0.254: v47.73,12.84 47.73,22.23 48.31,22.81 v49.99,22.81
N$18  (via drill 0.25)
  Top 0.102: U1.C5 v44.4,30 | v53.85,27.23 53.85,28.39 R52.1
  Bottom 0.102: v44.4,30 44.2,29.8 44.2,27.43 44.81,26.82 53.44,26.82 v53.85,27.23
N$19  (via drill 0.25)
  Top 0.102: U1.C1 49.4,29 v49.4,25.8 | v54.8,24.8 v54.8,22.8
  Top 0.254: R17.2 C16.1 v61.9,7.48 R23.2
  Bottom 0.102: v49.4,25.8 50,25.2 54.4,25.2 v54.8,24.8 | 56.6,22.4
  Bottom 0.254: v61.9,7.48 61.9,17.55 57.05,22.4 56.6,22.4 | v54.8,22.8 55.2,22.4 56.6,22.4
N$20
  Top 0.254: R4.1 12.95,36.02 13.01,35.97 15.95,35.97 16.26,36.27 16.8,36.27 IC4.7
N$21
  Top 0.254: R6.1 16.78,36.94 IC4.6
N$22  (via drill 0.25)
  Top 0.102: U1.B1 48.9,28.7 v48.9,23.4
  Top 0.254: R18.2 C17.1 61,12.84 R24.2 61.06,14.18 v61.06,19.61
  Bottom 0.254: v48.9,23.4 57.27,23.4 v61.06,19.61
N$23
  Top 0.254: IC4.11 18.87,33.49 R2.1
N$24  (via drill 0.25)
  Top 0.254: IC4.5 16.4,37.55 v16.05,37.9 | v16.05,33.53 16.91,33.53 R3.1
  Bottom 0.254: v16.05,37.9 v16.05,33.53
N$25
  Top 0.254: SV4.1 41.66,46.23 | 41.66,46.23 41.66,44.45 40.73,43.52 Q5.3 | R32.2 40.5,46.23 41.66,46.23
N$26
  Top 0.254: SV4.2 39.12,45.97 38.62,45.47 | 38.62,45.47 Q5.6 | R33.2 38.62,45.57 38.62,45.47
N$27  (via drill 0.25)
  Top 0.102: 35.48,9.55 IC5.10 | 35.31,20.83 Q10.6
  Top 0.254: v48.06,9.75 36.98,9.75 v36.78,9.55 35.48,9.55 | v36.37,20.83 35.31,20.83
  Bottom 0.254: SV2.1 50.8,7.01 v48.06,9.75 | v36.78,9.55 36.78,20.42 v36.37,20.83
N$28
  Top 0.102: U1.M11 39.6,38 39.6,39.4 39.02,39.98 34.29,39.98 32.26,42.01 28.85,42.01 28.5,42.37 28.5,43.48 28.49,43.48 Q7.1
N$29
  Top 1.27: D1.A 11.79,11.18 10.36,9.75 5.65,9.75 CN2.PWR1
N$30
  Top 0.102: U1.N7 43.2,40.35 45.21,42.37 Q4.1
N$31  (via drill 0.25)
  Top 0.102: v33.53,44.2 33.54,44.25 Q6.6
  Top 0.254: SV4.4 34.04,45.97 33.54,45.47 | 33.54,45.47 Q6.6 | R35.2 33.54,45.57 33.54,45.47
  Bottom 0.102: 33.02,44.15 33.07,44.2
  Bottom 0.254: SV5.4 64.77,29.21 64.77,30.99 63.96,31.8 63.96,37.49 60.55,40.89 33.68,40.89 33.02,41.55 33.02,44.15 | 33.07,44.2 v33.53,44.2
N$32
  Top 0.102: U1.N10 40.8,39.46 39.01,41.25 34.75,41.25 33.53,42.47 33.53,43.51 Q6.1
N$33
  Top 0.254: IC5.7 IC5.6 25.9,8.86 R48.1
N$34  (via drill 0.25)
  Top 0.102: U1.N8 42.4,40.16 44.81,42.57 44.81,44.09 44.91,44.2 v45.21,44.2 | Q4.4 v46.23,44.2
  Bottom 0.102: v46.23,44.2 v45.21,44.2
N$35
  Top 0.102: U1.M7 43.6,38 43.6,39.6 45.35,41.35 49.68,41.35 50.3,41.97 Q3.1
N$36
  Top 0.406: R56.1 LED7.A
N$37
  Top 0.254: QG1.3 34.06,37.08 R29.2
N$38  (via drill 0.25)
  Top 0.102: U1.N6 44,39.43 45.62,41.05 50.29,41.05 51.31,42.06 v51.31,42.88 | Q3.4 v51.31,44.2
  Bottom 0.102: v51.31,44.2 v51.31,42.88
N$39  (via drill 0.25)
  Top 0.254: SV4.5 31.5,46.23 | 31.5,46.23 31.5,44.45 30.57,43.52 v30.38,43.52 Q7.3 | R36.2 30.34,46.23 31.5,46.23
  Bottom 0.254: v30.38,43.52 30.38,41.15 31.24,40.28 60.3,40.28 63.3,37.29 63.3,31.6 63.5,31.39 SV5.1
N$40  (via drill 0.25)
  Top 0.102: U1.N9 41.6,40.19 v39.93,41.86 | Q6.4 v34.54,44.2 | v34.54,42.88 35.56,41.86 v38.51,41.86
  Bottom 0.102: v34.54,44.2 v34.54,42.88 | v38.51,41.86 v39.93,41.86
N$41  (via drill 0.25)
  Top 0.102: v28.3,39.73 28.09,39.73 27.84,39.98 27.84,43.69 28.35,44.2 28.35,44.76 Q7.6
  Top 0.254: SV4.6 28.96,45.97 28.57,45.59 | 28.57,45.59 28.46,45.47 Q7.6 | R37.2 28.43,45.59 28.57,45.59
  Bottom 0.254: SV5.3 62.23,29.21 62.23,32.82 62.69,33.27 62.69,37.03 59.99,39.73 v28.3,39.73
N$42
  Top 0.102: U1.M9 41.2,38 41.2,39.88 38.61,42.47 38.61,43.51 Q5.1
N$43
  Top 0.254: SV3.3 58.42,46.23 | 58.42,46.23 58.42,44.45 57.49,43.52 Q2.3 | R45.1 57.26,46.23 58.42,46.23
N$44
  Top 0.102: U1.N5 44.8,39.4 45.41,40.02 45.62,40.23 45.92,40.54 53.44,40.54 55.37,42.47 55.37,43.48 55.38,43.49 Q2.1
N$45  (via drill 0.25)
  Top 0.102: U1.N4 45.6,39.5 46.13,40.03 54.46,40.03 56.39,41.96 v56.39,42.88 | Q2.4 v56.39,44.2
  Bottom 0.102: v56.39,44.2 v56.39,42.88
N$46
  Top 0.254: SV3.4 55.88,45.97 55.5,45.59 | 55.5,45.59 55.38,45.47 Q2.6 | R44.1 55.36,45.59 55.5,45.59
N$47  (via drill 0.25)
  Top 0.254: Q9.1 12.51,23.86 v12.7,23.67 | v18.9,15.04 25.3,15.04 28.25,12.09 29.57,12.09 IC5.1
  Bottom 0.254: v12.7,23.67 12.7,21.23 v18.9,15.04
N$48
  Top 0.254: SV4.3 36.58,46.23 | 36.58,46.23 36.58,44.45 35.65,43.52 Q6.3 | R34.2 35.42,46.23 36.58,46.23
N$49
  Top 0.254: SV3.5 53.34,46.23 | 53.34,46.23 53.34,44.45 52.41,43.52 Q3.3 | R43.1 52.18,46.23 53.34,46.23
N$50  (via drill 0.25)
  Top 0.102: U1.C12 38.8,30 v37,30
  Top 0.254: IC7.1 25.43,27.23 26.2,28 v31,28
  Bottom 0.102: v31,28 32.8,28 34.8,30 v37,30
N$51
  Top 0.254: SV3.6 50.8,45.97 50.42,45.59 | 50.42,45.59 50.3,45.47 Q3.6 | R42.1 50.28,45.59 50.42,45.59
N$52  (via drill 0.25)
  Top 0.102: U1.B13 37.4,29.6 v37.1,29.3
  Top 0.254: IC7.2 26.7,26.7 27.4,27.4 v31.8,27.4
  Bottom 0.102: v31.8,27.4 33.2,27.4 35.2,29.4 37,29.4 v37.1,29.3
N$53  (via drill 0.25)
  Top 0.102: v20.83,46.99 20.18,47.64 R38.1 | v23.62,46.99 v23.61,46.99 Q11.3
  Bottom 0.102: v20.83,46.99 v23.62,46.99
N$54  (via drill 0.25)
  Top 0.102: R39.1 17.6,47.71 v17.6,48.4 | Q11.6 22.55,47.72 v22.55,48.5
  Bottom 0.102: v17.6,48.4 17.7,48.5 v22.55,48.5
N$55
  Top 0.254: SV3.1 63.5,46.23 | 63.5,46.23 63.5,44.45 62.57,43.52 Q1.3 | R47.1 62.34,46.23 63.5,46.23
N$56  (via drill 0.25)
  Top 0.102: 50.98,9.45 IC6.5
  Top 0.254: v55.37,9.45 50.98,9.45 | v50.19,18.49 44.5,18.49 44.09,18.9 44.09,19.75 Q12.3
  Bottom 0.254: SV2.4 58.42,4.98 55.58,7.82 55.58,9.25 v55.37,9.45 55.37,11.53 53.95,12.95 52.58,12.95 50.19,15.34 v50.19,18.49
N$57  (via drill 0.25)
  Top 0.102: 51.06,10.77 IC6.3 | 45.47,20.73 Q12.6
  Top 0.254: v52.93,10.77 51.06,10.77 | v49.48,20.12 49.28,20.32 47.04,20.32 46.74,20.32 46.24,20.82 Q12.6
  Bottom 0.254: SV2.3 55.88,6.5 54.97,7.42 54.97,8.74 v52.93,10.77 52.93,11.58 49.48,15.04 v49.48,20.12
N$58  (via drill 0.25)
  Top 0.102: U1.D2 v46.8,31.6 | v49.38,30.68 49.58,30.48 v52.53,30.48
  Top 0.254: R30.2 R59.2 59.48,31.9 v57,31.9
  Bottom 0.102: v46.8,31.6 47.6,30.8 48.79,30.8 48.91,30.68 v49.38,30.68 | v52.53,30.48 56.69,30.48 57,30.79 v57,31.9
N$59  (via drill 0.25)
  Top 0.102: U1.C4 v46,30 | v49.4,30 49.63,29.77 R53.1
  Bottom 0.102: v46,30 v49.4,30
N$60  (via drill 0.25)
  Top 0.102: U1.H6 43.6,34.8 41.4,34.8 41.2,35 41.2,35.4 41,35.6 v40.4,35.6 | v35.94,35.31 35.32,35.31 R29.1
  Top 0.254: R29.1 C24.1
  Bottom 0.102: v40.4,35.6 39.6,35.6 39.4,35.4 36.03,35.4 v35.94,35.31
N$61  (via drill 0.25)
  Top 0.102: U1.M8 42,38 42,40.5 v39.62,42.88 | Q5.4 v39.62,44.2
  Bottom 0.102: v39.62,44.2 v39.62,42.88
N$62
  Top 0.406: R3.2 LED2.C
N$63
  Top 0.254: 20.73,30.47 LED3.C
  Top 0.406: R5.2 LED3.C
N$64
  Top 0.254: SV3.2 60.96,45.97 60.46,45.47 | 60.46,45.47 Q1.6 | R46.1 60.46,45.57 60.46,45.47
N$65
  Top 0.254: SV3.8 45.72,45.97 45.34,45.59 | 45.34,45.59 45.22,45.47 Q4.6 | R40.1 45.2,45.59 45.34,45.59
N$66  (via drill 0.25)
  Top 0.102: U1.M12 38.8,38 37,38 35.63,39.37 33.98,39.37 32,41.35 v28.91,41.35 | v19.36,44.2 19.3,44.25 Q8.4
  Bottom 0.102: v28.91,41.35 27.58,42.67 21.13,42.67 19.61,44.2 v19.36,44.2
N$67  (via drill 0.25)
  Top 0.102: U1.D7 v42.8,31.6 | v35.4,27.6 35.4,29.13 R51.1
  Bottom 0.102: v42.8,31.6 39.6,28.4 38.8,28.4 37.8,27.4 35.6,27.4 v35.4,27.6
N$68  (via drill 0.25)
  Top 0.102: U1.M13 37,37.6 36.99,37.59 36.78,37.59 35.46,38.91 33.68,38.91 31.8,40.79 v28.3,40.79 | v18.29,42.67 v18.3,42.68 Q8.1
  Bottom 0.102: v28.3,40.79 26.77,42.32 20.88,42.32 20.52,42.67 v18.29,42.67
N$69  (via drill 0.25)
  Top 0.254: v21.34,37.59 20.31,37.59 IC4.16 | C3.2 16.56,39.42 16.66,39.32 v17.27,39.32
  Bottom 0.254: v21.34,37.59 19.1,39.83 17.78,39.83 v17.27,39.32
N$70  (via drill 0.25)
  Top 0.102: R22.2 44.81,7.48 44.81,7.42 | 46.74,7.42 C15.1 | U1.E4 v45.2,31.6 | v45.2,27.6 45.72,27.08 v45.72,22.25
  Top 0.254: 44.81,7.42 v45.72,7.42 46.74,7.42 | C15.1 R16.2
  Bottom 0.102: v45.2,31.6 44.6,31 44.6,30.6 45.2,30 v45.2,27.6
  Bottom 0.254: v45.72,7.42 v45.72,22.25
N$71  (via drill 0.25)
  Top 0.102: U1.D6 v43.6,31.6 | v49.4,35.6 52.81,39.01 R54.1
  Bottom 0.102: v43.6,31.6 43.6,32.4 45,33.8 45,34.8 45.2,35 48.2,35 48.8,35.6 v49.4,35.6
N$72
  Top 0.254: R1.1 R31.2 26.05,13.01 26.42,13.01 28.61,10.81 IC5.3
N$73  (via drill 0.25)
  Top 0.102: Q2.2 Q2.5 55.88,45.21 v56.24,45.57 | Q3.2 Q3.5 50.8,45.21 v51.16,45.57 | Q4.2 Q4.5 45.72,45.21 v46.08,45.57 | Q5.2 Q5.5 39.12,45.21 v39.47,45.57 | Q6.2 Q6.5 34.04,45.21 v34.39,45.57 | Q7.5 28.96,44.91 | Q7.5 Q7.2 | Q8.5 18.8,44.91 | Q8.5 Q8.2 | Q8.5 18.8,45.21 v19.15,45.57 | v29.31,45.57 28.96,45.21 Q7.5 | v61.32,45.57 60.96,45.21 Q1.5 Q1.2 v60.96,42.27 | C23.1 64.97,46.39 | v62.18,41.6 62.19,41.59 R57.2
  Top 0.254: R57.2 63.95,42.35 D8.C | 64.97,46.39 64.97,45.67 v65.08,45.57
  Bottom 0.102: v60.96,42.27 61.62,41.6 v62.18,41.6
  Bottom 0.254: v19.15,45.57 v29.31,45.57 v34.39,45.57 v39.47,45.57 v46.08,45.57 v51.16,45.57 v56.24,45.57 v61.32,45.57 v65.08,45.57
N$74  (via drill 0.25)
  Top 0.102: U1.C11 39.6,30 39.6,29.4 39.4,29.2 38,29.2 37.4,28.6 v36.2,28.6
  Top 0.254: IC7.3 27.96,26.16 28.4,26.6 v32.8,26.6
  Bottom 0.102: v32.8,26.6 33.4,26.6 35.4,28.6 v36.2,28.6
N$75  (via drill 0.25)
  Top 0.102: 35.58,10.67 IC5.12 35.4,10.77 | Q10.3 33.83,19.78
  Top 0.254: v48.97,10.46 37.29,10.46 36.94,10.81 IC5.12 | v33.83,11.07 34.14,10.77 35.4,10.77 | 33.83,19.78 v33.83,19.2
  Bottom 0.254: SV2.2 53.34,6.1 v48.97,10.46 | v33.83,19.2 v33.83,11.07
N$77  (via drill 0.25)
  Top 0.102: U1.E13 v36.8,32
  Top 0.254: v31.6,31.4 30.89,31.4 30.15,30.66 IC7.5
  Bottom 0.102: v36.8,32 33.8,32 33.2,31.4 v31.6,31.4
N$78  (via drill 0.25)
  Top 0.102: U1.D12 38.8,31.6 37.4,31.6 v37.2,31.4
  Top 0.254: IC7.6 27.96,29.43 28.2,29.2 v31.2,29.2
  Bottom 0.102: v31.2,29.2 32.4,29.2 34.2,31 36.2,31 36.6,31.4 v37.2,31.4
N$79  (via drill 0.25)
  Top 0.102: U1.D11 39.6,30.8 36.8,30.8 v36.6,30.6
  Top 0.254: IC7.7 26.7,29.11 27.2,28.6 v32,28.6
  Bottom 0.102: v32,28.6 32.6,28.6 34.4,30.4 36.4,30.4 v36.6,30.6
N$80
  Top 0.102: U1.K10 40.4,36.4 36.4,36.4 34.4,38.4 26.92,38.4 22.55,34.04 22.55,33.57 R56.2
N$81
  Top 0.406: R62.1 R63.2 22.75,1.89 23.88,0.76 23.88,0.71 28.65,0.71 SV1.2
N$82
  Top 0.102: Q11.5 Q11.2 23.11,45.87 23.37,45.62 23.77,45.62 24.13,45.26 24.13,44.04 Q13.3 24.5,42.63 R58.2
N$103  (via drill 0.25)
  Top 0.102: Q7.4 v29.46,44.2 | U1.L11 40.4,37.2 40.4,39.25 39.06,40.59 34.39,40.59 32.41,42.57 29.77,42.57 v29.46,42.88
  Bottom 0.102: v29.46,44.2 v29.46,42.88
NCONFIG
  Top 0.102: U1.E7 42.8,32.4 37.59,32.4 37.43,32.56 36.47,32.56 36.4,32.49 36.4,32.4 34.99,30.99 R50.1
RESET_N  (via drill 0.25)
  Top 0.102: C3.1 R49.1 | U1.B9 42,29.2 v42,27.2
  Top 0.254: R49.1 19.31,41.54 20.62,40.23 v23.27,40.23 | S1.4 12.38,45.72 C3.1 | v24.69,18.09 25.7,17.07 v26.72,17.07
  Bottom 0.254: SV1.3 33.02,17.17 | 33.02,17.17 33.02,22.65 33.1,22.73 33.1,23 37,26.9 41.7,26.9 v42,27.2 42.07,27.13 43.74,27.13 44.5,26.36 55.32,26.36 55.88,25.81 63.09,25.81 SV5.5 | v23.27,40.23 25.4,38.1 25.4,31.57 24.69,30.86 v24.69,18.09 | v26.72,17.07 26.82,17.17 33.02,17.17
RXD  (via drill 0.25)
  Top 0.102: U1.M5 45.2,38 v49.17,38 | v60.45,38.3 Q1.1 59.28,44.7 v59.18,44.7
  Top 0.254: v26.67,44.55 26.67,39.83 26.54,39.7 26.16,39.32 19.2,39.32 18.87,38.98 IC4.2
  Bottom 0.102: v26.67,44.55 27.13,45.01 58.98,45.01 59.18,44.81 v59.18,44.7 | v49.17,38 52.22,38 52.73,38.51 55.07,38.51 55.37,38.2 60.35,38.2 v60.45,38.3
SCL  (via drill 0.25)
  Top 0.254: SV4.10 18.8,45.97 18.41,45.59 | 18.41,45.59 18.3,45.47 Q8.6 | 18.41,45.59 18.27,45.59 R39.2 16.66,45.48 v16.66,43.08 | R61.2 18.8,26.72 19.61,27.53 v23.06,27.53
  Bottom 0.254: v23.06,27.53 23.06,36.68 v16.66,43.08
SCL_I  (via drill 0.25)
  Top 0.254: v24.13,5.08 60.96,5.08 SV2.6 | v59.18,10.16 58.42,10.16 57.77,10.81 IC6.12 56.73,10.77 55.78,10.77 55.47,11.07 v55.47,12.8 | Q14.3 54.19,19.44 v53.95,19.2 | R61.1 18.84,25.36 19.71,24.49 v22.86,24.49
  Bottom 0.254: v24.13,5.08 22.86,6.35 22.86,22.96 22.86,23.11 v22.86,24.49 | v59.18,10.16 59.18,6.86 SV2.6 | v53.95,19.2 53.95,14.33 v55.47,12.8
SDA  (via drill 0.25)
  Top 0.254: SV4.9 21.34,46.23 | 21.34,46.23 21.34,44.45 20.41,43.52 20.12,43.52 | 20.12,43.52 Q8.3 | R38.2 20.18,46.23 21.34,46.23 | 20.12,43.52 v20.12,41.96 | R60.2 23.61,26.66 v23.88,26.92
  Bottom 0.254: v23.88,26.92 23.88,38.2 v20.12,41.96
SDA_I  (via drill 0.25)
  Top 0.254: IC6.10 57.77,9.51 v57.91,9.65 | v24.89,6.1 58.67,6.1 v58.8,5.97 | Q14.6 v56.63,20.82 v56.64,20.83 | R60.1 23.61,25.36 v23.88,25.09
  Bottom 0.254: SV2.5 59.69,3.81 59.69,5.08 v58.8,5.97 57.91,6.86 v57.91,9.65 56.64,10.92 v56.64,20.83 | v24.89,6.1 24.03,6.96 24.03,23.11 23.88,23.27 v23.88,25.09
TXD  (via drill 0.25)
  Top 0.102: U1.M4 46,37.2 v49.2,37.2 | Q1.4 v61.47,44.2 | v61.47,42.88 61.47,37.8 60.87,37.2 v59.35,37.2
  Top 0.254: v27.48,44.55 27.23,44.3 27.23,39.42 26.52,38.71 25.2,38.71 23.39,36.9 IC4.15
  Bottom 0.102: v27.48,44.55 27.64,44.7 58.17,44.7 58.67,44.2 v61.47,44.2 v61.47,42.88 | v59.35,37.2 v49.2,37.2
VBUS_5V  (via drill 0.25)
  Top 0.254: 12.58,28.65 12.62,28.65
  Top 0.508: X1.1 6.17,39.7 4.17,37.69 4.17,35.26 5.38,34.04 5.38,32.61 5.99,32 10.26,32 11.68,30.58 11.68,29.55 12.58,28.65 Q9.3 | 12.62,28.65 C2.1
  Top 0.61: 5.99,32 5.28,31.29 5.28,30.84 v5.23,30.79 5.28,30.79 v5.84,30.23 5.79,30.28
  Bottom 0.61: TP6.TP 4.22,26.57 7.72,26.57 8.13,26.98 8.13,29.52 7.42,30.23 v5.84,30.23 5.28,30.79 v5.23,30.79 5.23,31.29 v5.49,31.55
VIN  (via drill 0.25)
  Top 0.406: v21.59,9.5 21.59,11.8 C19.1 R1.2
  Top 0.508: 18.46,11.62 21.41,11.62 C19.1
  Top 1.016: 18.46,11.62 14.53,15.54 v5.49,15.54 4.78,15.54 IC2.3
  Top 1.168: C27.+ 19.68,9.95 D1.C
  Top 1.27: D1.C 18.46,11.62
  Bottom 0.406: SV1.8 45.72,1.88 44.55,0.71 23.22,0.71 21.64,2.29 21.64,9.45 v21.59,9.5
  Bottom 1.27: TP4.TP 5.49,10.57 v5.49,15.54 5.59,15.65 v7.11,15.65 v8.94,15.65

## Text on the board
tPlace: RESET | D8 | D7 | D4 | D2 | TX | RX | AREF | D13 | D12 | SCL | SDA | GND | ~D9 | ~D6 | ~D5 | ~D3 | ~D11 | ~D10 | ISP | + | cfg_sel | TX | RX | 3.3 | D13 | 1 | - | 3 | 3.3 | 5 | 6 | 7 | 8 | 9 | 7v - 15v | IOREF | RST | 3.3v | 5v | GND | GND | Vin | A0 | A1 | A2 | A3 | A4 | A5 | 5 | IOREF / select | 3.3
bPlace: RoHS Compliant | D- | D+ | GND | aloriumtech.com/xlr8 | 5v | Designed and Manufactured in USA | Board Rev 2.2 | 02.2016 | Vin | GND
tNames: Released under the Creative Commons Attribution Share-Alike 4.0 License | https://creativecommons.org/licenses/by-sa/4/0/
